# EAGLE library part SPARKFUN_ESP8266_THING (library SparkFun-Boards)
SparkFun Thing Board The SparkFun ESP8266 Thing is a breakout and development board for the ESP8266 WiFi SoC SparkFun Products: SparkFun ESP8266 Thing
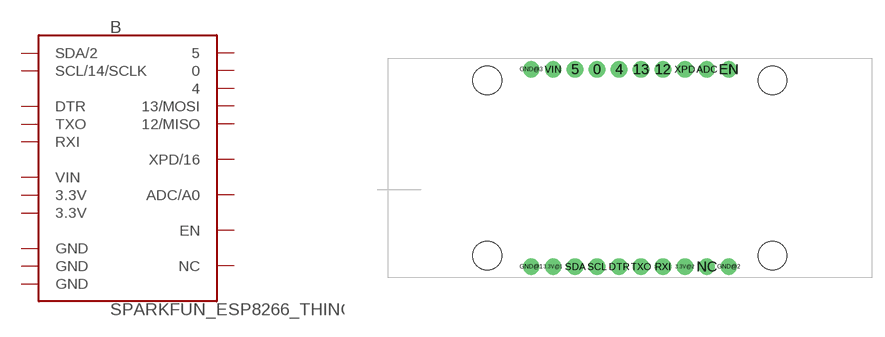
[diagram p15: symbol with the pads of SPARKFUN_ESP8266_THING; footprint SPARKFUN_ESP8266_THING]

Designator prefix B

## SPARKFUN_ESP8266_THING (SF_ID: WRL-13231)  [SPARKFUN_ESP8266_THING]
0  0
3.3V@1  3.3V  pwr
3.3V@2  3.3V  pwr
4  4
5  5
12  12/MISO
13  13/MOSI
ADC  ADC/A0
DTR  DTR
EN  EN  in
GND@1  GND  pwr
GND@2  GND  pwr
GND@3  GND  pwr
NC  NC  nc
RXI  RXI  in
SCL  SCL/14/SCLK
SDA  SDA/2
TXO  TXO  out
VIN  VIN  pwr
XPD  XPD/16

## Footprint SPARKFUN_ESP8266_THING (pad centres in mm)
SparkFun Thing Board Footprint Specifications: Pin count: 20 Pin pitch:0.1 inch Area: 2.2 x 1.0 inchees Example device(s): SparkFun Thing
drill 1.016 pad 1.88: 0 -2.54,11.43; 3.3V@1 -7.62,-11.43; 3.3V@2 7.62,-11.43; 4 0,11.43; 5 -5.08,11.43; 12 5.08,11.43; 13 2.54,11.43; ADC 10.16,11.43; DTR 0,-11.43; EN 12.7,11.43; GND@1 -10.16,-11.43; GND@2 12.7,-11.43; GND@3 -10.16,11.43; NC 10.16,-11.43; RXI 5.08,-11.43; SCL -2.54,-11.43; SDA -5.08,-11.43; TXO 2.54,-11.43; VIN -7.62,11.43; XPD 7.62,11.43
hole 3.302 at -15.24,-10.16
hole 3.302 at -15.24,10.16
hole 3.302 at 17.78,10.16
hole 3.302 at 17.78,-10.16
